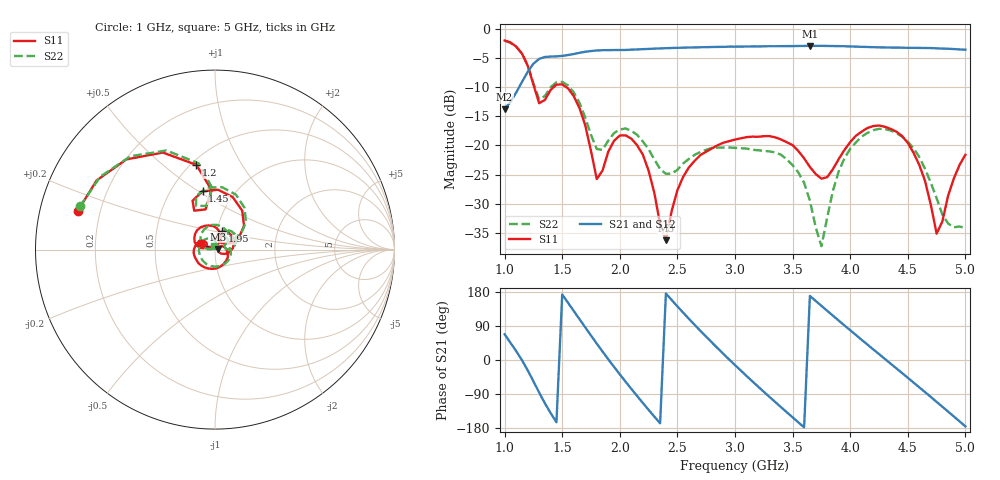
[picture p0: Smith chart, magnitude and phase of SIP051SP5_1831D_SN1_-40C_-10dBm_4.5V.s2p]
# GHz  S  dB  R  50
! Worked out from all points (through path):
!   81 points, 1 GHz to 5 GHz, reference 50 ohm
!   highest |S21| = -2.93 dB at 3.65 GHz (marker M1); lowest = -13.8 dB at 1 GHz (marker M2)
!   lowest |S11| = -36.2 dB at 2.4 GHz (marker M3), VSWR 1.03, Z = 51.5 + j0.288 ohm
!   |S11| at or under -10 dB: 1.257 GHz to 1.426 GHz (169.2 MHz wide, 12.6 % of centre); 1.535 GHz to end of sweep
!   |S22| runs from -37.3 to -2.0 dB; largest |S21 - S12| = 0.0022
!   S11 on the Smith chart (normalised r, x): 1 GHz: 0.12, +0.14; 1.2 GHz: 0.53, +0.66; 1.45 GHz: 0.71, +0.52; 1.95 GHz: 1.06, +0.22; 5 GHz: 0.86, +0.06
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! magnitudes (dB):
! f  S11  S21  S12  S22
! 1 GHz  -2.0  -13.8  -13.8  -2.0
! 1.2 GHz  -6.3  -7.4  -7.4  -6.2
! 1.3 GHz  -12.8  -5.2  -5.2  -12.1
! 1.45 GHz  -9.6  -4.7  -4.7  -9.2
! 1.7 GHz  -16.5  -3.9  -3.9  -15.2
! 1.8 GHz  -25.8  -3.7  -3.7  -20.6
! 1.95 GHz  -19.2  -3.6  -3.7  -17.9
! 2.2 GHz  -21.6  -3.5  -3.5  -19.3
! 2.35 GHz  -33.5  -3.4  -3.4  -24.0
! 2.4 GHz  -36.2  -3.3  -3.3  -24.9
! 2.6 GHz  -23.7  -3.2  -3.2  -22.3
! 3 GHz  -19.0  -3.1  -3.1  -20.4
! 3.4 GHz  -19.0  -3.0  -3.0  -21.6
! 3.65 GHz  -23.7  -2.9  -2.9  -29.4
! 3.7 GHz  -24.9  -2.9  -2.9  -34.0
! 3.75 GHz  -25.7  -2.9  -2.9  -37.3
! 3.85 GHz  -24.1  -3.0  -2.9  -27.8
! 4 GHz  -19.4  -3.0  -3.0  -20.6
! 4.35 GHz  -17.1  -3.2  -3.2  -17.4
! 4.6 GHz  -23.4  -3.3  -3.3  -22.0
! 4.75 GHz  -35.1  -3.4  -3.4  -29.0
! 5 GHz  -21.6  -3.6  -3.6  -34.2
